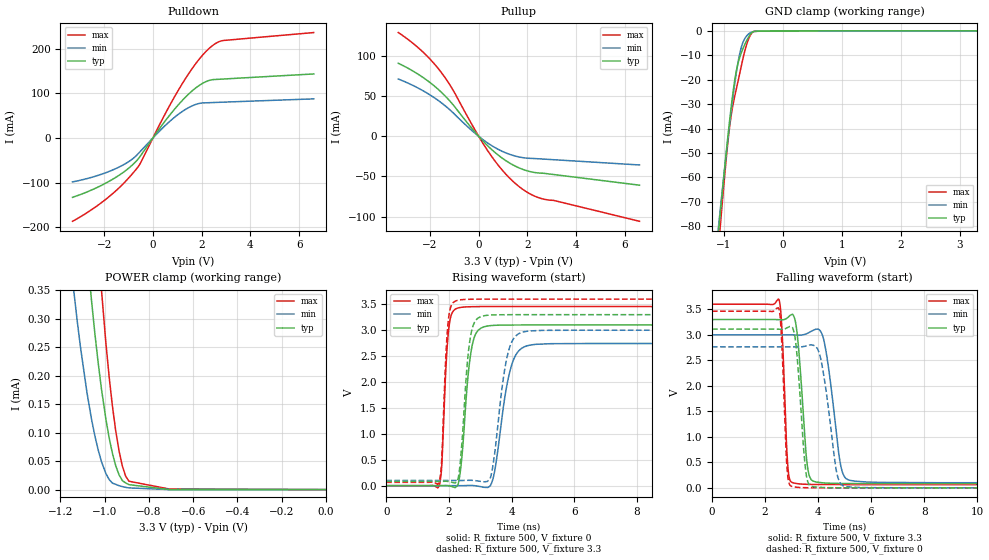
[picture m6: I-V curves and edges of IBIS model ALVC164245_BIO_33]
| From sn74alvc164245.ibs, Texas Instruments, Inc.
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[Model]   ALVC164245_BIO_33
Model_type  I/O
Vinl = 0.7
Vinh = 2
Enable   Active-Low
Vref =   0
Rref =   500
Cref =   30p
Vmeas =   1.5
| variable   typ   min   max
C_comp   8.5pF   NA   NA
| C_pullup   3.29pF   2.83pF   3.80pF
| C_pulldown   4.47pF   2.79pF   6.68pF
| C_tri-state   2.88pF   2.44pF   3.52pF
[Temperature Range]   40   100   -40
| Ambient temperature   25   85   -40
[Voltage range]   3.3   3   3.6
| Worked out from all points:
|   slope of the pulldown table from 0 to 0.495 V, typ, clamps not added: 13.2 ohm
|   slope of the pullup table from 0 to 0.495 V, typ, clamps not added: 32 ohm
|   GND clamp passes 1 mA (typ) near -0.54 V on its own axis
|   POWER clamp passes 1 mA (typ) near -1.18 V on its own axis
|   rising waveform, R_fixture 500, V_fixture 0: 20-80 % time 257ps typ, 411ps min, 159ps max; typ from 0 V to 3.1 V
|   falling waveform, R_fixture 500, V_fixture 3.3: 20-80 % time 258ps typ, 403ps min, 161ps max; typ from 3.3 V to 0.082 V
|   rising waveform, R_fixture 500, V_fixture 3.3: 20-80 % time 235ps typ, 363ps min, 149ps max; typ from 0.082 V to 3.3 V
|   falling waveform, R_fixture 500, V_fixture 0: 20-80 % time 256ps typ, 415ps min, 159ps max; typ from 3.11 V to 0 V
[GND Clamp]
| ALVC164245_BIO_33
|   Voltage   I(typ)   I(min)   I(max)
-3.3V     -724.5mA   -661.5mA   -819.8mA
-1.105V   -86.29mA   -83.67mA   -93.18mA
-1.08V    -79.83mA   -77.81mA   -85.86mA
-1.06V    -74.72mA   -73.17mA   -80.07mA
-915mV    -39.73mA   -41.03mA   -42.12mA
-865mV    -29.19mA   -30.91mA   -33.08mA
-805mV    -18.81mA   -19.95mA   -25.69mA
-750mV    -12.49mA   -11.73mA   -19.65mA
-690mV    -8.181mA   -5.715mA   -12.93mA
-545mV    -1.258mA   -688uA     -1.566mA
-420mV    -110.6uA   -127.7uA   -157uA
3.3V      15.97uA    12.63uA    25.22uA
[POWER Clamp]
| ALVC164245_BIO_33
|   Voltage   I(typ)   I(min)   I(max)
-3.3V     48.51mA    36.53mA    69.64mA
-1.145V   760.3uA    367.6uA    1.302mA
-1.125V   645uA      298.8uA    1.119mA
-1.08V    419.2uA    170.2uA    755.6uA
-1.06V    334.2uA    124.8uA    616.1uA
-1.015V   178.2uA    49.76uA    353.2uA
-980mV    91.47uA    17.83uA    199.1uA
-950mV    41.93uA    9.227uA    103.2uA
-920mV    15.8uA     5.245uA    41.37uA
-890mV    8.657uA    2.99uA     14.66uA
-710mV    128.9nA    111.5nA    1.203uA
-48.03fV  45.95pA    1.365nA    344.9pA
[Pulldown]
| ALVC164245_BIO_33
|   Voltage   I(typ)   I(min)   I(max)
-3.3V     -132.9mA   -98.33mA   -186.5mA
-2.505V   -116.2mA   -87.96mA   -160.1mA
-1.8V     -97.07mA   -74.96mA   -131.4mA
-1.12V    -73.07mA   -57.28mA   -96.89mA
-660mV    -50.38mA   -38.26mA   -68.24mA
-490mV    -38.45mA   -28.51mA   -54mA
435mV     33.08mA    24.23mA    46.88mA
1.17V     81.89mA    57.92mA    118.4mA
1.86V     116.1mA    76.74mA    173.7mA
2.43V     130.3mA    79.23mA    206.1mA
2.89V     132mA      80.17mA    218.2mA
6.6V      143.3mA    87.53mA    235.9mA
[Pullup]
| ALVC164245_BIO_33
|   Voltage   I(typ)   I(min)   I(max)
-3.3V     90.96mA    71.35mA    129.1mA
-2.37V    75mA       58.15mA    107.2mA
-1.605V   56.9mA     43.37mA    82.22mA
-1.095V   40.83mA    30.52mA    59.67mA
-135mV    4.712mA    3.405mA    7.045mA
435mV     -13.75mA   -9.703mA   -20.88mA
1.055V    -29.13mA   -19.9mA    -45.17mA
1.67V     -39.51mA   -25.81mA   -62.92mA
2.115V    -43.99mA   -27.47mA   -71.82mA
2.565V    -45.92mA   -28.2mA    -77.44mA
3.065V    -47.55mA   -29.13mA   -79.74mA
6.6V      -60.88mA   -35.7mA    -105.8mA
[Ramp]
| ALVC164245_BIO_33
| variable   typ   min   max
dV/dt_r   1.88/2.64E-10   1.67/4.17E-10   2.10/1.65E-10
dV/dt_f   1.99/2.73E-10   1.81/4.26E-10   2.18/1.72E-10
R_load = 500
[Rising Waveform]
| ALVC164245_BIO_33
R_fixture =   500
C_fixture =   0
L_fixture =   0
V_fixture =   0
V_fixture_min = 0
V_fixture_max = 0
|   Time   V(typ)   V(min)   V(max)
0s        99.03pV    3.812nV    31.44nV
1.685ns   -117.7uV   1.753uV    -7.125mV
2.005ns   -3.356mV   -37.65uV   3.074V
2.42ns    585.7mV    293.7uV    3.444V
2.645ns   2.309V     4.079mV    3.452V
2.87ns    2.944V     -4.518mV   3.455V
3.4ns     3.092V     117.2mV    3.457V
4.07ns    3.1V       2.441V     3.457V
4.765ns   3.101V     2.728V     3.457V
50ns      3.101V     2.743V     3.457V
[Falling Waveform]
| ALVC164245_BIO_33
R_fixture =   500
C_fixture =   0
L_fixture =   0
V_fixture =   3.3
V_fixture_min = 3
V_fixture_max = 3.6
|   Time   V(typ)   V(min)   V(max)
0s        3.3V       3V         3.6V
2.525ns   3.297V     3V         3.691V
2.64ns    3.293V     3V         3.081V
2.88ns    3.349V     3V         312.5mV
3.24ns    2.883V     2.995V     80.73mV
3.685ns   213.7mV    3.054V     68.11mV
4.18ns    99.06mV    2.973V     65.2mV
4.875ns   86.13mV    393.4mV    64.28mV
5.435ns   83.74mV    129.6mV    64.09mV
50ns      81.97mV    99.96mV    63.94mV
[Rising Waveform]
| ALVC164245_BIO_33
R_fixture =   500
C_fixture =   0
L_fixture =   0
V_fixture =   3.3
V_fixture_min = 3
V_fixture_max = 3.6
|   Time   V(typ)   V(min)   V(max)
0s        81.96mV    99.95mV    63.93mV
1.685ns   81.86mV    99.95mV    64.98mV
1.99ns    79.98mV    99.92mV    3.231V
2.385ns   593.3mV    100.1mV    3.588V
2.61ns    2.506V     103.3mV    3.596V
2.805ns   3.137V     99.56mV    3.598V
3.325ns   3.293V     151.6mV    3.6V
3.895ns   3.299V     2.579V     3.6V
4.565ns   3.3V       2.986V     3.6V
50ns      3.3V       3V         3.6V
[Falling Waveform]
| ALVC164245_BIO_33
R_fixture =   500
C_fixture =   0
L_fixture =   0
V_fixture =   0
V_fixture_min = 0
V_fixture_max = 0
|   Time   V(typ)   V(min)   V(max)
0s        3.113V     2.764V     3.463V
2.515ns   3.11V      2.764V     3.52V
2.845ns   3.142V     2.764V     294.5mV
3.155ns   2.862V     2.762V     14.72mV
3.54ns    313.4mV    2.781V     3.469mV
3.82ns    22.47mV    2.796V     1.567mV
4.145ns   8.171mV    2.419V     704.3uV
4.72ns    2.102mV    262.9mV    238.4uV
5.05ns    1.191mV    24.42mV    150.8uV
50ns      7.549uV    12.98uV    6.405uV
